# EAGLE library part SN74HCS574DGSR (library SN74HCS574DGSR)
Flip-Flops Octal edge-triggered D-type flip-flops w Source: Datasheet
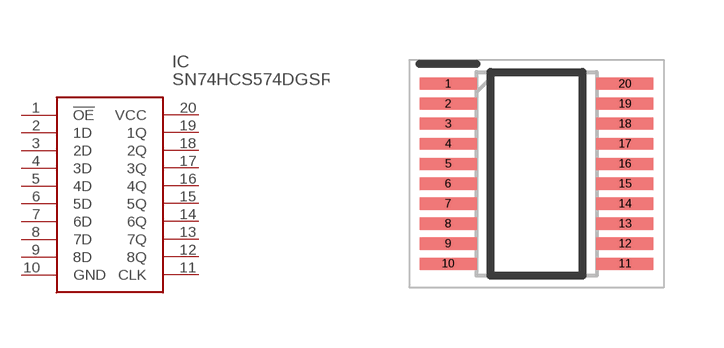
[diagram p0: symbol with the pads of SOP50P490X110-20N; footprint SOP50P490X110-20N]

Designator prefix IC

## SN74HCS574DGSR (Description: Flip-Flops Octal edge-triggered D-type flip-flops w; Height: 1.1mm; Manufacturer_Name: Texas Instruments; Manufacturer_Part_Number: SN74HCS574DGSR)  [SOP50P490X110-20N]
1  !OE
2  1D
3  2D
4  3D
5  4D
6  5D
7  6D
8  7D
9  8D
10  GND
11  CLK
12  8Q
13  7Q
14  6Q
15  5Q
16  4Q
17  3Q
18  2Q
19  1Q
20  VCC

## Footprint SOP50P490X110-20N (pad centres in mm)
DGS0020A
smd 1.425 x 0.3: 1 -2.212,2.25; 2 -2.212,1.75; 3 -2.212,1.25; 4 -2.212,0.75; 5 -2.212,0.25; 6 -2.212,-0.25; 7 -2.212,-0.75; 8 -2.212,-1.25; 9 -2.212,-1.75; 10 -2.212,-2.25; 11 2.212,-2.25; 12 2.212,-1.75; 13 2.212,-1.25; 14 2.212,-0.75; 15 2.212,-0.25; 16 2.212,0.25; 17 2.212,0.75; 18 2.212,1.25; 19 2.212,1.75; 20 2.212,2.25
